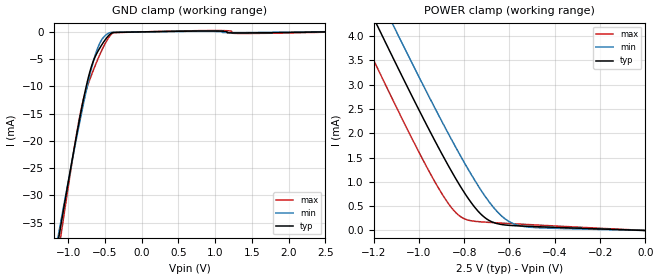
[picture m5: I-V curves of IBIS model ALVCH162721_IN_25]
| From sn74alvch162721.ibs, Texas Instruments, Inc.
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[Model]   ALVCH162721_IN_25
Model_type  Input
Vinl = 0.7
Vinh = 1.7
| variable   typ   min   max
C_comp   1.84pF   1.57pF   2.07pF
[Temperature Range]   40   100   -40
| Ambient temperature   25   85   -40
[Voltage range]   2.5   2.3   2.7
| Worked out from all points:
|   GND clamp passes 1 mA (typ) near -0.47 V on its own axis
|   POWER clamp passes 1 mA (typ) near -0.83 V on its own axis
[GND Clamp]
| ALVCH162721_IN_25
|   Voltage   I(typ)   I(min)   I(max)
-2.5V     -153.2mA   -143.6mA   -168.7mA
-1.15V    -39.47mA   -38.43mA   -41.94mA
-1.115V   -36.66mA   -35.85mA   -38.77mA
-1.085V   -34.27mA   -33.64mA   -36.06mA
-940mV    -22.97mA   -23.19mA   -23.22mA
-840mV    -15.61mA   -16.31mA   -15.24mA
-730mV    -8.578mA   -9.318mA   -9.607mA
-665mV    -5.593mA   -5.765mA   -7.269mA
-590mV    -3.421mA   -2.659mA   -4.792mA
-460mV    -821.1uA   -306.8uA   -1.275mA
-375mV    -100.8uA   -82.47uA   -137.6uA
2.5V      35.46pA    35.81uA    -58.91uA
[POWER Clamp]
| ALVCH162721_IN_25
|   Voltage   I(typ)   I(min)   I(max)
-2.5V     17.35mA    17.92mA    16.64mA
-1.26V    4.955mA    5.626mA    4.095mA
-1.18V    4.182mA    4.857mA    3.313mA
-1.11V    3.512mA    4.192mA    2.639mA
-1.08V    3.229mA    3.909mA    2.355mA
-940mV    1.94mA     2.615mA    1.09mA
-845mV    1.129mA    1.778mA    407.8uA
-795mV    748uA      1.36mA     232.5uA
-725mV    330.7uA    823.9uA    177uA
-625mV    116.2uA    259uA      149.5uA
-510mV    84.14uA    67.22uA    120.3uA
-31.15fV  6.662pA    8.896pA    6.889pA
